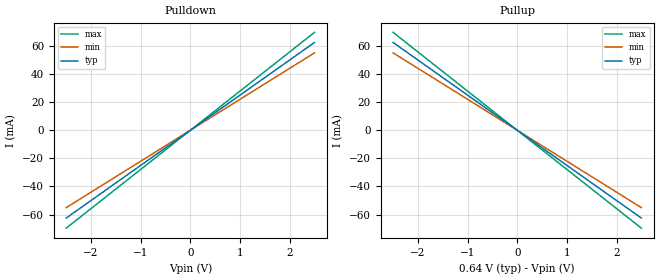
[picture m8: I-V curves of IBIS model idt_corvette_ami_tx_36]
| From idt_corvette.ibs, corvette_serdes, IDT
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|   model   idt_corvette_ami_tx_36
[Model] idt_corvette_ami_tx_36
Model_type Output
C_comp 400f 400f 400f
Cref = 0
[Model Spec]
Vmeas 0. 0. 0.
Vref 0. 0. 0.
[Temperature Range]  25 100 0
[Voltage Range] .64 .643 .531
[Algorithmic Model]
Executable Windows_VisualStudio5_32 idt_corvette_tx.dll   idt_corvette_tx.ami
Executable Windows_ver_64   idt_corvette_tx_64.dll   idt_corvette_tx.ami
Executable Linux_gcc4.1.2_32   idt_corvette_tx.linux.so   idt_corvette_tx.ami
Executable Linux_gcc3.2.3_64   idt_corvette_tx_64.linux.so idt_corvette_tx.ami
[End Algorithmic Model]
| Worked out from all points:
|   slope of the pulldown table from 0 to 0.096 V, typ, clamps not added: 40 ohm
|   slope of the pullup table from 0 to 0.096 V, typ, clamps not added: 40 ohm
[Pulldown]
-2.5V     -62.5mA    -55.1mA    -69.69mA
0V        0A         0A         0A
2.5V      62.5mA     55.1mA     69.69mA
[Pullup]
-2.5V     62.5mA     55.1mA     69.69mA
0V        0A         0A         0A
2.5V      -62.5mA    -55.1mA    -69.69mA
[Ramp]
dV/dt_r .213/22.4p .202/25.41p .186/20.089p
dV/dt_f .213/22.4p .202/25.41p .186/20.089p
